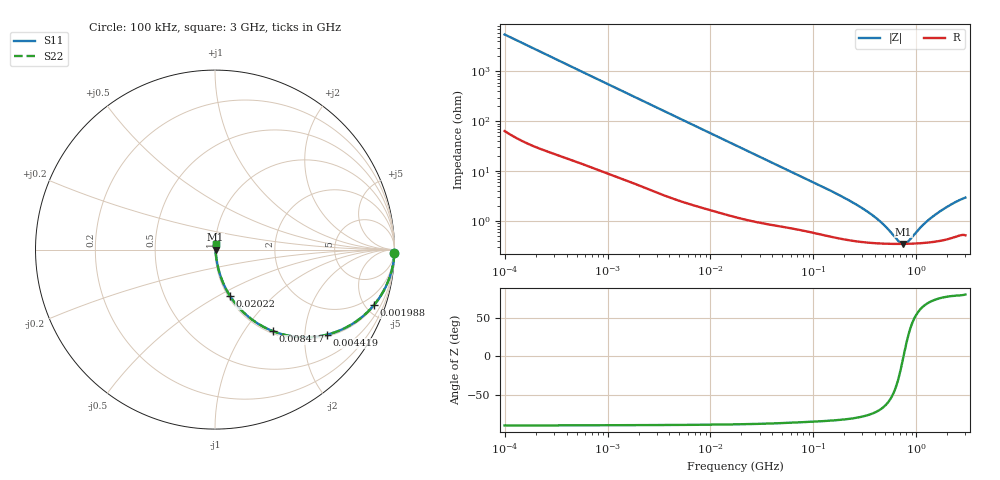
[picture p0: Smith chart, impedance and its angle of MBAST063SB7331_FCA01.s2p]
! MBAST063SB7331_FCA01  S-PARAMETER MODEL  ( Standard Model )
! Model Generated by TAIYO YUDEN Corporation (http://www.ty-top.com)
! Version 2.0
! TAIYO YUDEN Control No. 231201
! Copyright(c) 2020 TAIYO YUDEN CO.,LTD. All Rights Reserved.
! Product Description (link to TY-COMPAS)
! https://ds.yuden.co.jp/TYCOMPAS/or/detail?pn=MBAST063SB7331KFCA01&u=M
! Products Name : Multilayer Ceramic Capacitors
! Characteristics :
!  Capacitance : 330 [pF] , Rated Voltage : 25 [V] , TCC : X7R
!  Case Size : 0.6 x 0.3 / 0.024 x 0.012 [mm/inch] , Thickness : 0.3 / 0.012 [mm/inch]
!  (Conditions: Temperature = 25 [degC] , DC Bias Voltage = 0 [V])
! External Node Assignments :
!  1  o---| |---o  2
! GND o---------o GND
! Frequency Range : 100kHz  -  3GHz  [ 401 STEP ]
# MHZ S RI R 50
! Freq[MHz].  S11 Real  S11 Imag  S21 Real  S21 Imag  S12 Real  S12 Imag  S22 Real  S22 Imag
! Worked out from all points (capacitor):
!   401 points, 100 kHz to 3 GHz, reference 50 ohm
!   read as one part in series: C = 288 pF near 105.3 kHz
!   lowest |Z| = 346 mohm at 746 MHz (marker M1)
!   series resonance near 751.9 MHz, so ESL is about 160 pH
!   S11 on the Smith chart (normalised r, x): 100 kHz: open; 1.988 MHz: 1.10, -5.69; 4.419 MHz: 1.06, -2.58; 8.417 MHz: 1.04, -1.36; 20.22 MHz: 1.02, -0.57; 3 GHz: 1.01, +0.06
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0.1  0.9995 -0.0181  0.000534 0.0181  0.000534 0.0181  0.9995 -0.0181
0.562235  0.9886 -0.0994  0.0114 0.0994  0.0114 0.0994  0.9886 -0.0994
1.156955  0.9564 -0.1962  0.0436 0.1962  0.0436 0.1962  0.9564 -0.1962
1.987766  0.8855 -0.3094  0.1145 0.3094  0.1145 0.3094  0.8855 -0.3094
3.161081  0.7592 -0.4177  0.2408 0.4177  0.2408 0.4177  0.7592 -0.4177
4.419184  0.6221 -0.4743  0.3779 0.4743  0.3779 0.4743  0.6221 -0.4743
8.417093  0.322 -0.4542  0.678 0.4542  0.678 0.4542  0.322 -0.4542
12.07428  0.1933 -0.3798  0.8067 0.3798  0.8067 0.3798  0.1933 -0.3798
17.7727  0.1047 -0.2887  0.8953 0.2887  0.8953 0.2887  0.1047 -0.2887
20.21703  0.0848 -0.2601  0.9152 0.2601  0.9152 0.2601  0.0848 -0.2601
41.60216  0.0271 -0.1361  0.9729 0.1361  0.9729 0.1361  0.0271 -0.1361
97.38194  0.00945 -0.0601  0.9906 0.0601  0.9906 0.0601  0.00945 -0.0601
294.964  0.00407 -0.0178  0.9959 0.0178  0.9959 0.0178  0.00407 -0.0178
412.3589  0.00365 -0.0105  0.9963 0.0105  0.9963 0.0105  0.00365 -0.0105
547.5153  0.00348 -0.00534  0.9965 0.00534  0.9965 0.00534  0.00348 -0.00534
672.8816  0.00344 -0.00184  0.9966 0.00184  0.9966 0.00184  0.00344 -0.00184
745.9503  0.00344 -0.00013  0.9966 0.00013  0.9966 0.00013  0.00344 -0.00013
826.9535  0.00346 0.00158  0.9965 -0.00158  0.9965 -0.00158  0.00346 0.00158
1156.079  0.00364 0.00733  0.9964 -0.00733  0.9964 -0.00733  0.00364 0.00733
1535  0.00398 0.0128  0.996 -0.0128  0.996 -0.0128  0.00398 0.0128
2259.438  0.00504 0.0216  0.995 -0.0216  0.995 -0.0216  0.00504 0.0216
3000  0.00595 0.0286  0.9941 -0.0286  0.9941 -0.0286  0.00595 0.0286
